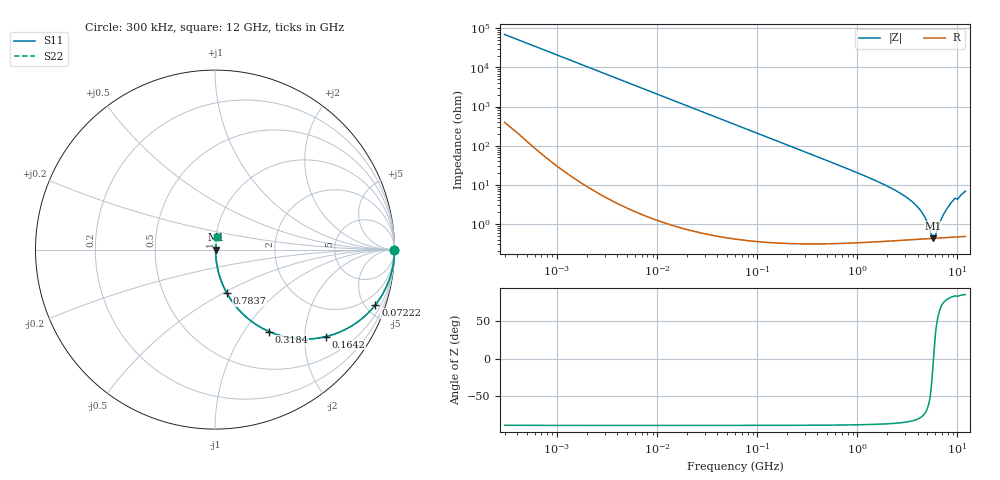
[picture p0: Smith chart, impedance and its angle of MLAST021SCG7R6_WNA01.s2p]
! MLAST021SCG7R6_WNA01  S-PARAMETER MODEL  ( General Type )
! Model Generated by TAIYO YUDEN Corporation (http://www.ty-top.com)
! Version 1.0
! TAIYO YUDEN Control No. 220901
! Copyright(c) 2022 TAIYO YUDEN CO.,LTD. All Rights Reserved.
! Product Description (link to TY-COMPAS)
! https://ds.yuden.co.jp/TYCOMPAS/or/detail?pn=MLAST021SCG7R6CWNA01&u=M
! Products Name : Multilayer Ceramic Capacitors
! Characteristics :
!  Capacitance : 7.6 pF , Rated Voltage : 25V , TCC : CG / C0G
!  Case Size : 0.25 x 0.125 / 0.0098 x 0.0049 [mm/inch] , Thickness : 0.125 / 0.0049 [mm/inch]
!  (Conditions: Temperature = 25 degC , DC Bias Current/Voltage = 0A / 0V)
! External Node Assignments :
!  1  o---| |---o  2
! GND o---------o GND
! Frequency Range : 0.3MHz  -  12000MHz  [ 401 STEP ]
# MHz S RI R 50
! Freq[MHz].  S11 Real  S11 Imag  S21 Real  S21 Imag  S12 Real  S12 Imag  S22 Real  S22 Imag
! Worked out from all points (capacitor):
!   401 points, 300 kHz to 12 GHz, reference 50 ohm
!   read as one part in series: C = 7.6 pF near 316.3 kHz
!   lowest |Z| = 432 mohm at 5.715 GHz (marker M1)
!   series resonance near 5.768 GHz, so ESL is about 100 pH
!   S11 on the Smith chart (normalised r, x): 300 kHz: open; 72.22 MHz: 1.01, -5.80; 164.2 MHz: 1.01, -2.55; 318.4 MHz: 1.01, -1.31; 783.7 MHz: 1.01, -0.52; 12 GHz: 1.01, +0.14
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0.3  1 -0.00143  1.01e-05 0.00143  1.01e-05 0.00143  1 -0.00143
1.769972  0.9999 -0.00845  7.92e-05 0.00845  7.92e-05 0.00845  0.9999 -0.00845
10.44266  0.9975 -0.0497  0.00251 0.0497  0.00251 0.0497  0.9975 -0.0497
27.10171  0.9834 -0.1273  0.0166 0.1273  0.0166 0.1273  0.9834 -0.1273
60  0.9239 -0.2646  0.0761 0.2646  0.0761 0.2646  0.9239 -0.2646
72.22496  0.8933 -0.308  0.1067 0.308  0.1067 0.308  0.8933 -0.308
107.4644  0.791 -0.4057  0.209 0.4057  0.209 0.4057  0.791 -0.4057
164.1901  0.6186 -0.4845  0.3814 0.4845  0.3814 0.4845  0.6186 -0.4845
318.4019  0.3015 -0.4566  0.6985 0.4566  0.6985 0.4566  0.3015 -0.4566
353.9943  0.2589 -0.4354  0.7411 0.4354  0.7411 0.4354  0.2589 -0.4354
783.7017  0.0669 -0.2439  0.9331 0.2439  0.9331 0.2439  0.0669 -0.2439
2088.533  0.0111 -0.0857  0.9889 0.0857  0.9889 0.0857  0.0111 -0.0857
3107.553  0.00611 -0.0471  0.9939 0.0471  0.9939 0.0471  0.00611 -0.0471
4050.141  0.0047 -0.0257  0.9953 0.0257  0.9953 0.0257  0.0047 -0.0257
4747.894  0.00434 -0.0138  0.9957 0.0138  0.9957 0.0138  0.00434 -0.0138
5420.343  0.00425 -0.00412  0.9957 0.00412  0.9957 0.00412  0.00425 -0.00412
5715.274  0.00427 -0.000511  0.9957 0.000511  0.9957 0.000511  0.00427 -0.000511
6026.253  0.00431 0.00284  0.9957 -0.00284  0.9957 -0.00284  0.00431 0.00284
7064.448  0.00462 0.0145  0.9954 -0.0145  0.9954 -0.0145  0.00462 0.0145
8281.503  0.00537 0.0291  0.9946 -0.0291  0.9946 -0.0291  0.00537 0.0291
9207.246  0.00634 0.0416  0.9937 -0.0416  0.9937 -0.0416  0.00634 0.0416
12000  0.00941 0.0679  0.9906 -0.0679  0.9906 -0.0679  0.00941 0.0679
